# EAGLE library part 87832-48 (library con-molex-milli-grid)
HEADER
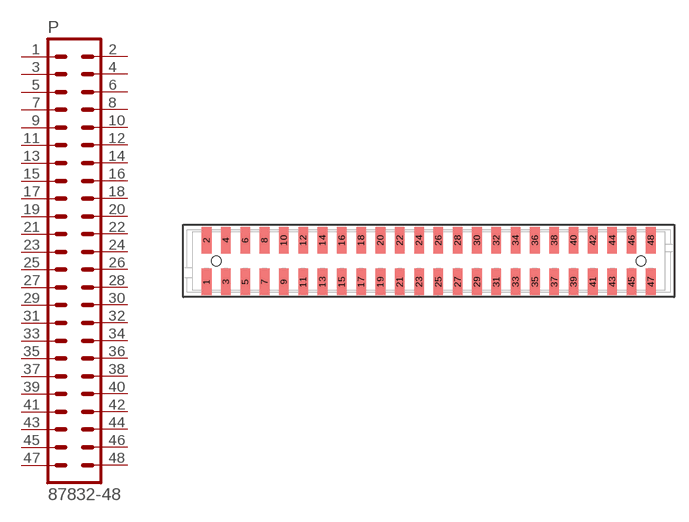
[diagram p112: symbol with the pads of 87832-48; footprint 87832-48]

Designator prefix P

## 87832-48  [87832-48]
1  1  pas
2  2  pas
3  3  pas
4  4  pas
5  5  pas
6  6  pas
7  7  pas
8  8  pas
9  9  pas
10  10  pas
11  11  pas
12  12  pas
13  13  pas
14  14  pas
15  15  pas
16  16  pas
17  17  pas
18  18  pas
19  19  pas
20  20  pas
21  21  pas
22  22  pas
23  23  pas
24  24  pas
25  25  pas
26  26  pas
27  27  pas
28  28  pas
29  29  pas
30  30  pas
31  31  pas
32  32  pas
33  33  pas
34  34  pas
35  35  pas
36  36  pas
37  37  pas
38  38  pas
39  39  pas
40  40  pas
41  41  pas
42  42  pas
43  43  pas
44  44  pas
45  45  pas
46  46  pas
47  47  pas
48  48  pas

## Footprint 87832-48 (pad centres in mm)
HEADER SMD Dual Row, Shrouded, Vertical
smd 1 x 2.75: 1 -23,-2.15; 2 -23,2.15; 3 -21,-2.15; 4 -21,2.15; 5 -19,-2.15; 6 -19,2.15; 7 -17,-2.15; 8 -17,2.15; 9 -15,-2.15; 10 -15,2.15; 11 -13,-2.15; 12 -13,2.15; 13 -11,-2.15; 14 -11,2.15; 15 -9,-2.15; 16 -9,2.15; 17 -7,-2.15; 18 -7,2.15; 19 -5,-2.15; 20 -5,2.15; 21 -3,-2.15; 22 -3,2.15; 23 -1,-2.15; 24 -1,2.15; 25 1,-2.15; 26 1,2.15; 27 3,-2.15; 28 3,2.15; 29 5,-2.15; 30 5,2.15; 31 7,-2.15; 32 7,2.15; 33 9,-2.15; 34 9,2.15; 35 11,-2.15; 36 11,2.15; 37 13,-2.15; 38 13,2.15; 39 15,-2.15; 40 15,2.15; 41 17,-2.15; 42 17,2.15; 43 19,-2.15; 44 19,2.15; 45 21,-2.15; 46 21,2.15; 47 23,-2.15; 48 23,2.15
hole 1 at -22,0
hole 1 at 22,0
